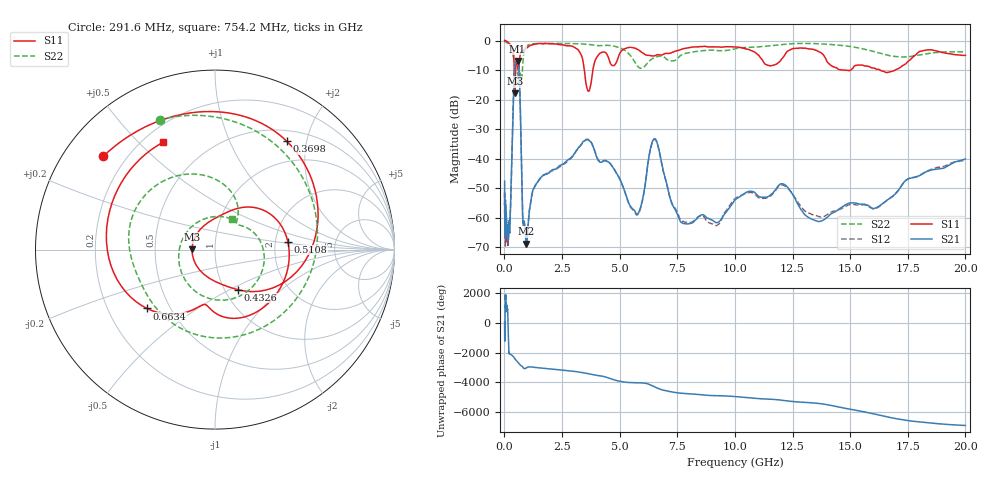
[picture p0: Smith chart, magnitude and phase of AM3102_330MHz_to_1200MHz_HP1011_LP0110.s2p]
! Date/Time: Tue, Sep 11, 2018 5:20 PM
! Network Analyzer: Agilent Technologies E8362B Rev: A.07.50.63
! Sweep from 0.010 to 20.000 GHz, 1601 Points, Sweep Type: LOG
! Power Supply: 4.949 V, 0.001 A
# Hz S DB R 50
!freq MagS11 AngS11 MagS21 AngS21 MagS12 AngS12 MagS22 AngS22
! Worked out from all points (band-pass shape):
!   1601 points, 10 MHz to 20 GHz, reference 50 ohm
!   highest |S21| = -6.92 dB at 572.5 MHz (marker M1); lowest = -68.8 dB at 951.8 MHz (marker M2)
!   |S21| within 3 dB of the highest: 433.4 MHz to 632.7 MHz (199.2 MHz wide, 37.4 % of centre)
!   lowest |S11| = -17.9 dB at 453.6 MHz (marker M3), VSWR 1.29, Z = 38.7 + j0.0639 ohm
!   |S11| at or under -10 dB: 3.469 GHz to 3.837 GHz (368.1 MHz wide, 10.1 % of centre); 14.67 GHz to 15.02 GHz (352.6 MHz wide, 2.38 % of centre); 16.3 GHz to 16.96 GHz (657.3 MHz wide, 3.95 % of centre)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
!   |S22| runs from -14.8 to -0.2 dB; largest |S21 - S12| = 0.0073
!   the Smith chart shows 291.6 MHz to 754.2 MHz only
!   S11 on the Smith chart (normalised r, x): 291.6 MHz: 0.12, +0.36; 369.8 MHz: 0.66, +1.67; 432.6 MHz: 1.15, -0.55; 510.8 MHz: 2.35, +0.25; 663.4 MHz: 0.37, -0.33; 754.2 MHz: 0.28, +0.59
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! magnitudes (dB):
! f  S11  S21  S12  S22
! 10 MHz  0.0  -47.7  -53.3  -0.2
! 35.55 MHz  0.0  -63.5  -65.8  -0.3
! 47.5 MHz  0.0  -59.3  -54.7  -0.4
! 126.4 MHz  -0.4  -64.5  -67.9  -0.8
! 291.6 MHz  -1.8  -50.3  -50.6  -2.1
! 369.8 MHz  -2.8  -25.3  -25.4  -4.9
! 432.6 MHz  -11.8  -10.0  -10.1  -6.6
! 447.2 MHz  -17.3  -8.5  -8.5  -6.9
! 453.6 MHz  -17.9  -8.0  -8.1  -6.9
! 510.8 MHz  -7.8  -7.2  -7.2  -6.1
! 572.5 MHz  -8.3  -6.9  -7.0  -9.7
! 663.4 MHz  -6.0  -15.4  -15.5  -11.0
! 754.2 MHz  -3.5  -46.3  -46.3  -14.2
! 951.8 MHz  -2.6  -68.8  -69.1  -2.0
! 1.59 GHz  -1.1  -46.3  -46.3  -1.0
! 3.634 GHz  -17.1  -33.7  -33.5  -1.3
! 5.652 GHz  -2.6  -57.8  -58.0  -7.2
! 6.487 GHz  -5.2  -33.4  -33.6  -5.9
! 7.92 GHz  -2.5  -62.1  -61.6  -4.2
! 12.03 GHz  -6.3  -48.5  -48.9  -1.4
! 13.74 GHz  -4.2  -61.2  -59.9  -1.1
! 20 GHz  -5.0  -40.1  -40.7  -3.8
